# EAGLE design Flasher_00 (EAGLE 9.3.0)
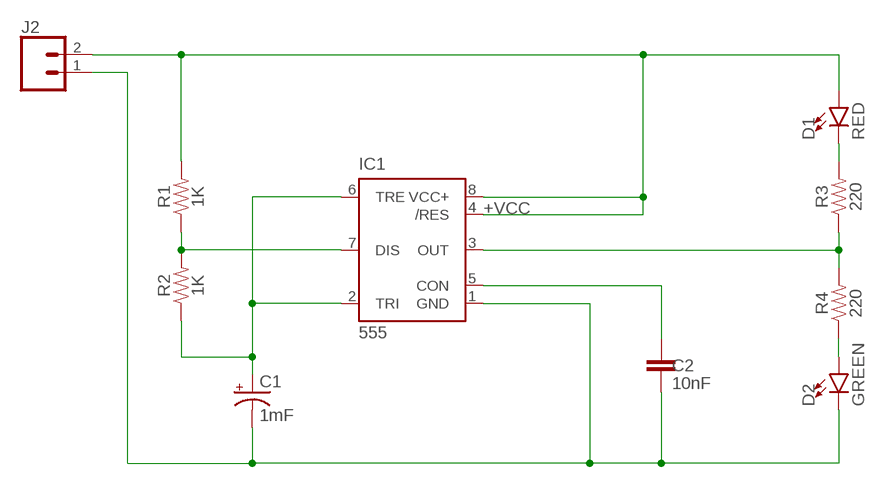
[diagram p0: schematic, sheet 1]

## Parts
C1  1mF  1000UF-RADIAL-5MM-25V-20%  [CPOL-RADIAL-5MM-10MM]
C2  10nF  10NF-PTH-10MM-10000V-1-%  [CAP-PTH-10MM]
D1  RED  LED5MM  [LED_5MM]
D2  GREEN  LED5MM  [LED_5MM]
IC1  555  555P  [DIP08]
J2  CONN_025MM  [SCREWTERMINAL-5MM-2]
R1  1K  10OHM-HORIZ-1/4W-1%  [AXIAL-0.3]
R2  1K  10OHM-HORIZ-1/4W-1%  [AXIAL-0.3]
R3  220  10OHM-HORIZ-1/4W-1%  [AXIAL-0.3]
R4  220  10OHM-HORIZ-1/4W-1%  [AXIAL-0.3]

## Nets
+VCC: D1.A IC1.4(/RES) IC1.8(VCC+) J2.2 R1.P$2
GND: C1.- C2.2 D2.K(C) IC1.1(GND) J2.1
N$1: D2.A R4.P$1
N$2: IC1.3(OUT) R3.P$1 R4.P$2
N$3: D1.K(C) R3.P$2
N$6: IC1.7(DIS) R1.P$1 R2.P$2
N$7: C2.1 IC1.5(CON)
N$8: C1.+ IC1.2(TRI) IC1.6(TRE) R2.P$1

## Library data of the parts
C1 = SparkFun-Capacitors:1000UF: 1,000µF/1mF ceramic capacitors; PROD_ID: CAP-09538
C2 = SparkFun-Capacitors:10NF: 0.01uF/10nF/10,000pF ceramic capacitors; PROD_ID: CAP-09321
D1 D2 = SparkFun-LED:LED: LED (Generic)
IC1 = SparkFun-IC-Special-Function:555: General purpose bipolar Timer Datasheet SparkFun Products SparkFun SparkPunk Sequencer Kit (KIT-12707) Storefront Component: 555 Timer (COM-09273) Two parts valid for production: VFP: IC-11930 (M7555 PTH) VFP: IC-09173 (555 PTH) - Preferred; PROD_ID: IC-09173; PROD_ID_ALT: IC-09173
J2 = SparkFun-Connectors:CONN_02: Multi connection point. Often used as Generic Header-pin footprint for 0.1 inch spaced/style header connections; SF_SKU: PRT-08432
R1-R4 = SparkFun-Resistors:10OHM: 10Ω resistor; PROD_ID: RES-12180; VALUE: 10

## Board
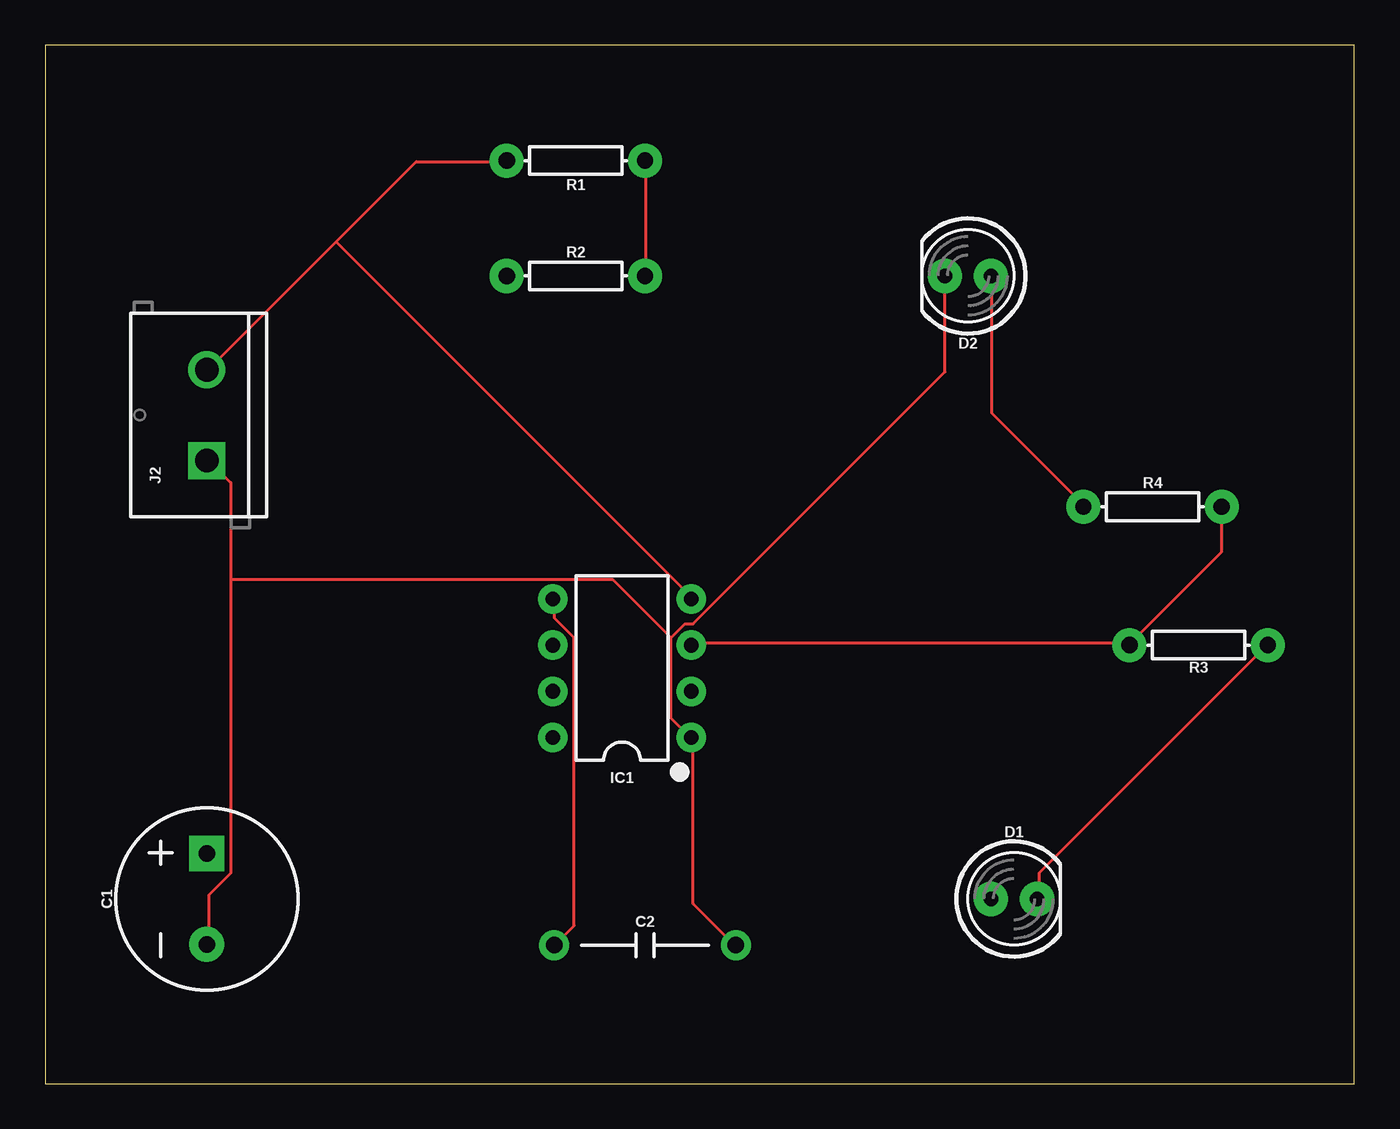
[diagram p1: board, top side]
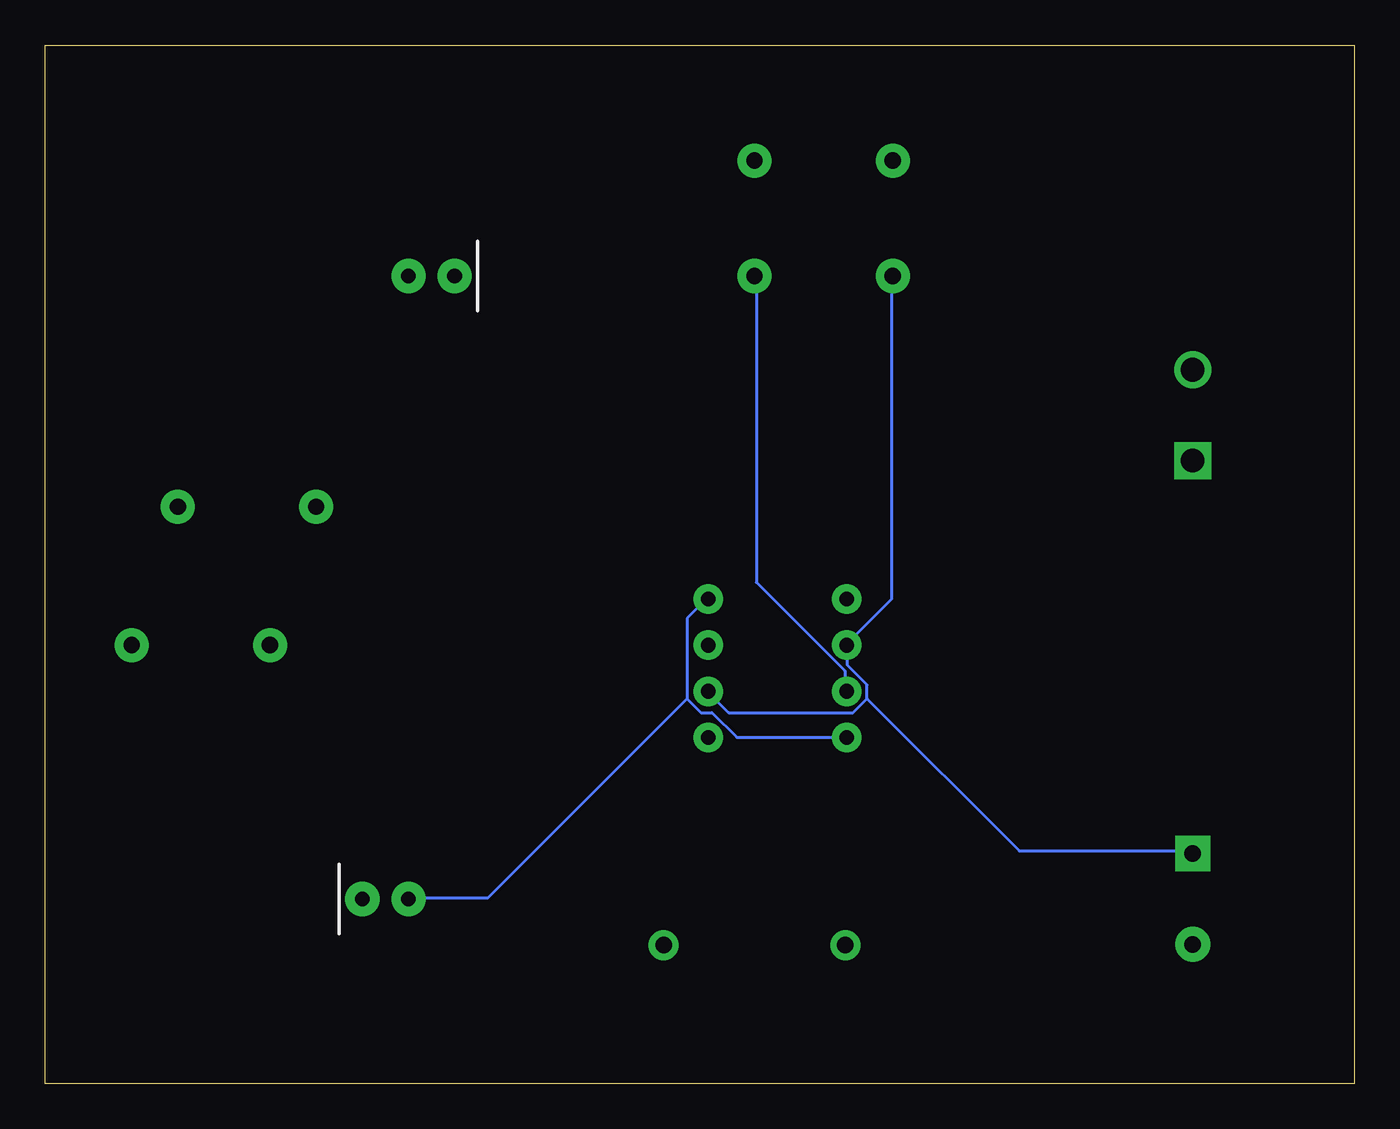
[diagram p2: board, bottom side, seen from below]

Size 72.06 x 57.14 mm. Coordinates in mm from the lower left corner, seen from the top.
Outline: 0,0 72.06,0 72.06,57.14 0,57.14 0,0
Copper layers (1*16): Top 0.035mm / dielectric 1.5mm / Bottom 0.035mm
Design rules "default": minimum track width 6mil, minimum drill 0.35mm, track to track 6mil, track to pad 6mil, pad to pad 6mil, via to via 6mil, smd to smd 6mil, copper to edge 40mil, drill to drill 6mil, minimum pad ring 10mil, minimum via ring 8mil, stop-mask expansion 4mil, vias tented up to drill 0mil, thermal gap 10mil

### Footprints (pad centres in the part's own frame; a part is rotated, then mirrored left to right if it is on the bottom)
CPOL-RADIAL-5MM-10MM = drill 0.9 pad 1.93 square: + 2.5,0 | drill 0.9 pad 1.93: - -2.5,0
CAP-PTH-10MM = drill 0.9 pad 1.651: 1 -5,0; 2 5,0
LED_5MM = drill 0.813 pad 1.88: A -1.27,0; K 1.27,0
DIP08 = drill 0.813 pad 1.626: 1 -3.81,-3.81; 2 -1.27,-3.81; 3 1.27,-3.81; 4 3.81,-3.81; 5 3.81,3.81; 6 1.27,3.81; 7 -1.27,3.81; 8 -3.81,3.81
SCREWTERMINAL-5MM-2 = drill 1.3 pad 2.032 square: 1 0,0 | drill 1.3 pad 2.032: 2 5,0
AXIAL-0.3 = drill 0.9 pad 1.88: P$1 -3.81,0; P$2 3.81,0

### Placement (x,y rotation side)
C1  8.89,10.16 90 top
C2  33.02,7.62 0 top
D1  53.34,10.16 0 top
D2  50.8,44.45 180 top
IC1  31.75,22.86 90 top
J2  8.89,34.29 90 top
R1  29.21,50.8 180 top
R2  29.21,44.45 0 top
R3  63.5,24.13 0 top
R4  60.96,31.75 0 top

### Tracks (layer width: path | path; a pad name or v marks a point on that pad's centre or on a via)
+VCC
  Top 0.152: 16,46.33 8.99,39.32 J2.2 | 16,46.33 20.42,50.75 25.3,50.75 R1.P$2 | 16,46.33 35.66,26.67 IC1.4
  Bottom 0.152: IC1.8 33.98,19.05 35.36,20.42 35.97,20.42 36.73,21.18 | 36.73,21.18 36.73,25.6 35.66,26.67 IC1.4 | 36.73,21.18 47.7,10.21 51.97,10.21 D1.A
GND
  Top 0.152: 10.21,27.74 10.21,33.07 8.99,34.29 J2.1 | 10.21,27.74 10.21,11.58 8.99,10.36 8.99,7.77 C1.- | C2.2 37.95,7.62 35.66,9.91 35.66,19.05 IC1.1 35.51,19.05 34.44,20.12 34.44,24.54 | D2.K 49.53,39.17 35.66,25.3 35.2,25.3 34.44,24.54 | 10.21,27.74 31.24,27.74 34.44,24.54
N$1
  Top 0.152: D2.A 52.12,44.35 52.12,36.88 57.15,31.85 R4.P$1
N$2
  Top 0.152: IC1.3 35.66,24.23 59.59,24.23 R3.P$1 59.74,24.23 64.77,29.26 R4.P$2
N$3
  Top 0.152: D1.K 54.71,10.21 54.71,11.58 67.21,24.08 R3.P$2
N$6
  Top 0.152: R1.P$1 33.07,50.75 33.07,44.5 R2.P$2
  Bottom 0.152: IC1.7 28.04,21.64 28.04,22.71 32.92,27.58 32.92,44.35 R2.P$2
N$7
  Top 0.152: IC1.5 28.04,26.67 28.04,25.6 29.11,24.54 29.11,8.69 28.04,7.62 C2.1
N$8
  Bottom 0.152: 26.82,21.18 26.82,21.95 27.89,23.01 27.89,24.08 IC1.6 27.89,24.23 25.45,26.67 25.45,44.35 R2.P$1 | 26.82,21.18 27.58,20.42 34.44,20.42 35.51,21.49 IC1.2 | 26.82,21.18 18.44,12.8 8.99,12.8 C1.+

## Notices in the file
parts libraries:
SparkFun-IC-Special-Function: Licensing: Creative Commons ShareAlike 4.0 International - https://creativecommons.org/licenses/by-sa/4.0
